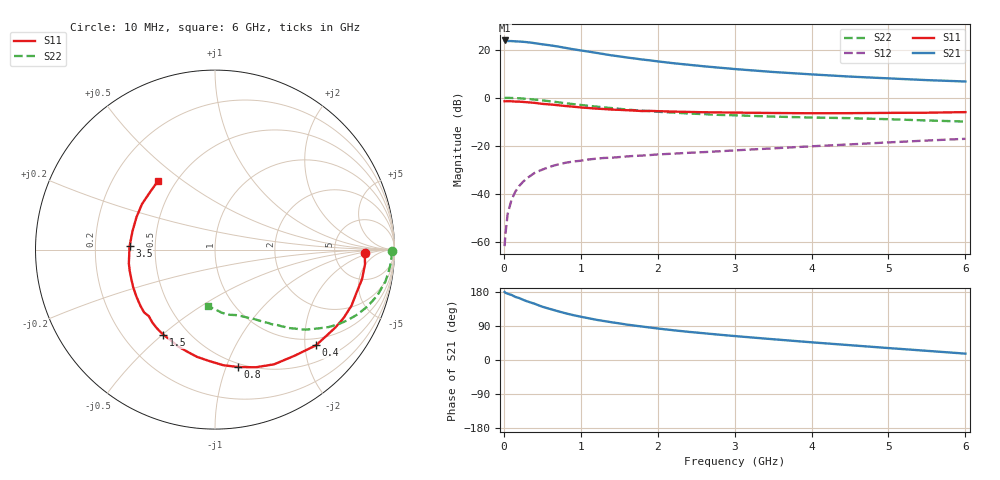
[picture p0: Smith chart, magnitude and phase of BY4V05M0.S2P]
! SIEMENS Small Signal Semiconductors
! BFY420
! Si NPN RF SIEGET Grounded Emitter Transistor in MICRO-X
! VCE = 4 V  IC = 5 mA
! Common Emitter S-Parameters:  October  1996
# GHz  S  MA  R  50
!  f  S11  S21  S12  S22
! GHz  MAG  ANG  MAG  ANG  MAG  ANG  MAG  ANG
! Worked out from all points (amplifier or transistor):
!   36 points, 10 MHz to 6 GHz, reference 50 ohm
!   highest |S21| = 23.8 dB at 10 MHz (marker M1)
!   |S21| within 3 dB of that: start of sweep to 785.6 MHz
!   unconditionally stable (mu >= 1): start of sweep to 10.57 MHz; 3.175 GHz to end of sweep
!   at 250 MHz: K = 0.17, MSG = 29.2 dB, |S12| = -35.1 dB
!   at 1.4 GHz: K = 0.53, MSG = 21.3 dB, |S12| = -25.1 dB
!   at 6 GHz: K = 1.13, MAG = 9.8 dB, |S12| = -17.2 dB
!   S11 on the Smith chart (normalised r, x): 10 MHz: 11, -2; 400 MHz: 0.84, -2.25; 800 MHz: 0.47, -1.10; 1.5 GHz: 0.37, -0.50; 3.5 GHz: 0.35, +0.02; 6 GHz: 0.40, +0.41
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0.01  0.8371 -1.4  15.49 179.6  0.0008 33.0  0.9856 -0.5
0.02  0.8352 -2.3  15.39 177.4  0.0014 56.0  0.9833 -1.0
0.05  0.8399 -5.6  15.09 174.9  0.0038 73.1  0.9841 -2.6
0.1  0.8354 -11.4  15.02 171.7  0.0074 78.7  0.9799 -5.4
0.15  0.8244 -16.8  14.85 166.5  0.011 78.0  0.9727 -8.1
0.2  0.8222 -22.3  14.7 163.4  0.0144 75.5  0.9662 -10.6
0.3  0.7986 -33.0  14.27 155.0  0.0208 71.0  0.9405 -15.7
0.4  0.7755 -43.4  13.62 148.4  0.0269 66.1  0.9078 -20.3
0.5  0.7392 -53.1  12.86 140.6  0.0315 62.8  0.873 -24.4
0.6  0.719 -62.7  12.28 134.7  0.0362 58.9  0.8363 -28.1
0.8  0.6669 -78.8  10.86 123.4  0.0437 52.4  0.7645 -34.4
0.9  0.6462 -85.8  10.17 118.5  0.0465 50.1  0.7311 -36.8
1.1  0.6058 -99.6  9.083 110.2  0.0512 46.8  0.6742 -41.4
1.3  0.5769 -111.0  8.053 102.9  0.0551 43.8  0.6239 -44.8
1.5  0.555 -121.3  7.225 96.7  0.0575 41.9  0.5824 -47.8
1.8  0.523 -134.8  6.206 88.2  0.0618 39.8  0.5337 -51.6
2.2  0.5104 -149.0  5.204 78.6  0.0678 38.8  0.4865 -56.0
2.8  0.4898 -165.9  4.198 66.8  0.0759 37.4  0.4355 -61.7
3.5  0.4765 177.8  3.413 54.8  0.0874 36.5  0.4016 -67.7
4.5  0.4733 157.6  2.735 39.1  0.1057 33.4  0.3721 -77.4
5.5  0.4835 138.3  2.308 24.2  0.1272 28.5  0.3331 -89.9
6  0.4973 129.7  2.162 16.8  0.1382 25.4  0.3163 -97.4
